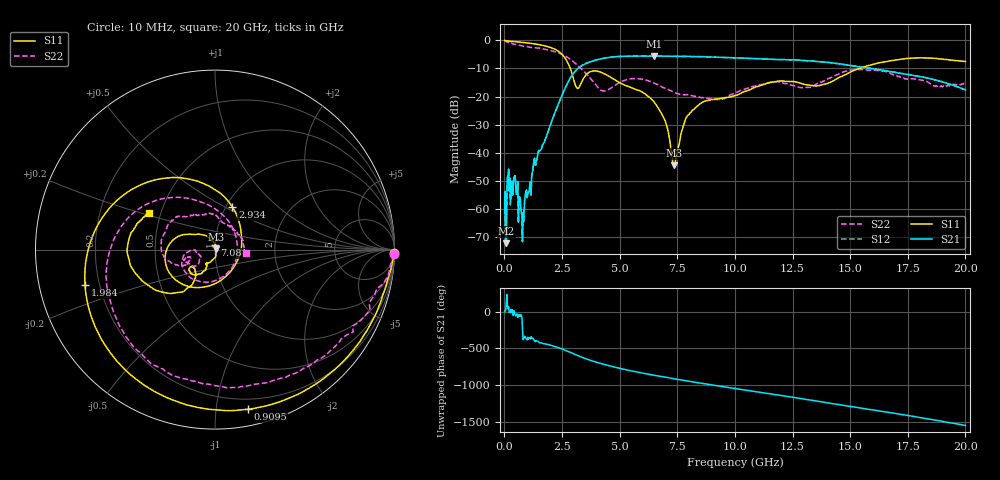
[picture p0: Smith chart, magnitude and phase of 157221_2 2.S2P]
!  2-Port S-parameters saved by WinCal
! VAR MeasName=S-Parameters (CALIBRATED_DATA) read from VNA (N5242A)
! VAR MeasDate=2015-5-26 16:47:24
! VAR NAME=157221_2 2
! VAR FILENAME=157221_2 2.S2P
! VAR DATE=2015-5-26 16:47:24
! VAR PHYS_PORTS=1,2
# Hz S DB R 50
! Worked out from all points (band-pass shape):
!   801 points, 10 MHz to 20 GHz, reference 50 ohm
!   highest |S21| = -5.61 dB at 6.507 GHz (marker M1); lowest = -72.3 dB at 84.96 MHz (marker M2)
!   |S21| within 3 dB of the highest: 3.447 GHz to 14.75 GHz (11.31 GHz wide, 124 % of centre)
!   lowest |S11| = -44.5 dB at 7.356 GHz (marker M3), VSWR 1.01, Z = 50.6 + j0.065 ohm
!   |S11| at or under -10 dB: 2.862 GHz to 15.41 GHz (12.55 GHz wide, 137 % of centre)
!   |S22| runs from -21.1 to 0.0 dB; largest |S21 - S12| = 0.0095
!   S11 on the Smith chart (normalised r, x): 10 MHz: open; 909.5 MHz: 0.12, -1.22; 1.984 GHz: 0.14, -0.13; 2.934 GHz: 1.07, +0.54; 7.081 GHz: 1.00, +0.05; 20 GHz: 0.43, +0.21
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1e7  -0.04 -1.1  -61.59 -1.9  -67.37 77.9  -0.04 -1.6
8.49625e7  -0.17 -8.6  -72.29 140.0  -73.29 135.4  -0.39 -11.5
2.348875e8  -0.30 -21.6  -49.11 -3.8  -49.11 -4.6  -0.85 -25.1
4.847625e8  -0.48 -43.1  -50.20 -53.0  -50.09 -52.9  -1.45 -45.6
7.0965e8  -0.66 -62.0  -59.54 -61.6  -60.23 -66.8  -1.88 -62.8
9.0955e8  -0.84 -78.3  -55.29 5.7  -55.38 3.5  -2.15 -77.1
1.984012e9  -2.48 -164.6  -30.46 -95.1  -30.46 -95.2  -3.64 -150.9
2.558725e9  -5.53 134.4  -18.43 -154.6  -18.42 -154.8  -5.20 169.4
2.933538e9  -11.84 67.7  -12.45 155.5  -12.44 155.4  -7.18 142.3
3.358325e9  -14.72 -85.8  -9.01 98.2  -8.98 98.0  -10.30 113.8
4.532738e9  -12.75 163.7  -6.09 -16.1  -6.10 -16.5  -17.43 -39.6
5.457275e9  -16.63 144.7  -5.62 -83.8  -5.63 -84.1  -13.71 -129.0
6.50675e9  -22.13 118.3  -5.61 -147.5  -5.62 -147.6  -15.26 -171.5
6.681662e9  -24.15 112.5  -5.63 -157.5  -5.63 -157.6  -15.91 -173.4
7.081462e9  -31.54 90.3  -5.66 -179.3  -5.65 -179.6  -17.41 -178.0
7.356325e9  -44.46 6.2  -5.69 165.9  -5.66 165.6  -18.47 -178.7
8.055975e9  -25.84 -96.3  -5.74 129.2  -5.72 128.9  -19.52 -171.7
1.0005e10  -19.60 -116.0  -6.23 32.7  -6.23 32.2  -18.80 -140.9
1.192904e10  -14.44 -134.4  -6.83 -58.8  -6.82 -59.6  -14.77 -162.2
1.335332e10  -16.05 -140.7  -7.41 -129.0  -7.35 -129.3  -16.44 -157.4
1.667666e10  -7.39 -153.4  -11.05 65.7  -11.00 65.2  -11.50 136.3
2e10  -7.51 151.2  -17.58 -111.3  -17.67 -113.0  -15.34 -5.7
